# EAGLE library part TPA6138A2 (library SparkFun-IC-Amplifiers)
Headphone driver amp Differential to single-ended audio amplifier. Datasheet SparkFun Products SparkFun Purpletooth Jamboree - BC127 Development Board (WRL-11924)
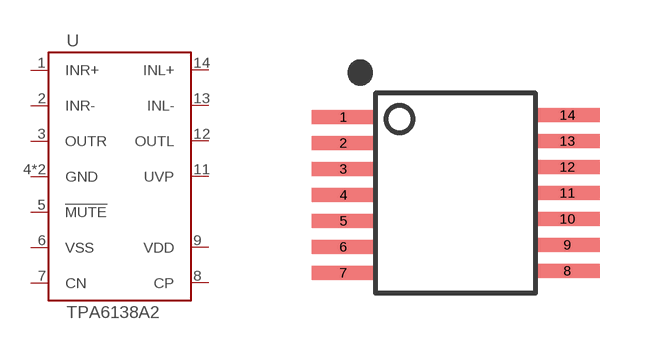
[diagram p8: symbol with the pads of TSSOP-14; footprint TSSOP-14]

Designator prefix -

## TPA6138A2 (PROD_ID: IC-11779; VALUE: TPA6138A2)  [TSSOP-14]
1  INR+
2  INR-
3  OUTR
4  GND
5  !MUTE
6  VSS
7  CN
8  CP
9  VDD
10  GND
11  UVP
12  OUTL
13  INL-
14  INL+

## Footprint TSSOP-14 (pad centres in mm)
smd 1.6 x 0.35: 1 -2.8,1.9; 2 -2.8,1.25; 3 -2.8,0.6; 4 -2.8,-0.05; 5 -2.8,-0.7; 6 -2.8,-1.35; 7 -2.8,-2; 8 2.8,-1.95; 9 2.8,-1.3; 10 2.8,-0.65; 11 2.8,0; 12 2.8,0.65; 13 2.8,1.3; 14 2.8,1.95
